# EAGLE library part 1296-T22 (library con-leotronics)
1.27mm SINGLE ROW FEMALE SOCKET Source: http://www.leotronics.co.uk/Conexcon/Data%20Sheets/sec.%20A/1296ing.pdf
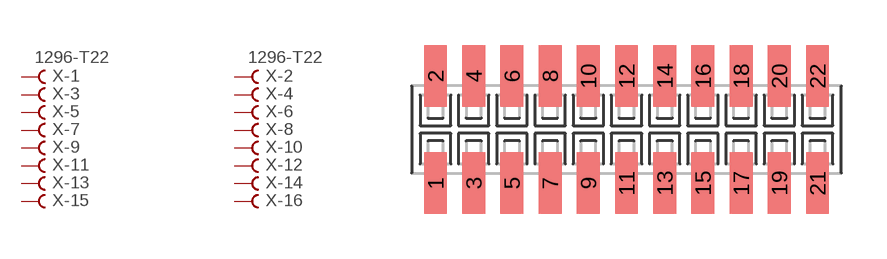
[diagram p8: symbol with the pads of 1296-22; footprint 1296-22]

Designator prefix X; gates -1=FVAL -2=FVAL -3=F -4=F -5=F -6=F -7=F -8=F -9=F -10=F -11=F -12=F -13=F -14=F -15=F -16=F -17=F -18=F -19=F -20=F -21=F -22=F

## 1296-T22 (OC_FARNELL: unknown; OC_NEWARK: unknown)  [1296-22]
1  -1:B  pas
2  -2:B  pas
3  -3:B  pas
4  -4:B  pas
5  -5:B  pas
6  -6:B  pas
7  -7:B  pas
8  -8:B  pas
9  -9:B  pas
10  -10:B  pas
11  -11:B  pas
12  -12:B  pas
13  -13:B  pas
14  -14:B  pas
15  -15:B  pas
16  -16:B  pas
17  -17:B  pas
18  -18:B  pas
19  -19:B  pas
20  -20:B  pas
21  -21:B  pas
22  -22:B  pas

## Footprint 1296-22 (pad centres in mm)
1.27mm SINGLE ROW FEMALE SOCKET Source: http://www.leotronics.co.uk/Conexcon/Data%20Sheets/sec.%20A/1296ing.pdf
smd 0.76 x 2.05: 1 -6.35,-1.78; 2 -6.35,1.78; 3 -5.08,-1.78; 4 -5.08,1.78; 5 -3.81,-1.78; 6 -3.81,1.78; 7 -2.54,-1.78; 8 -2.54,1.78; 9 -1.27,-1.78; 10 -1.27,1.78; 11 0,-1.78; 12 0,1.78; 13 1.27,-1.78; 14 1.27,1.78; 15 2.54,-1.78; 16 2.54,1.78; 17 3.81,-1.78; 18 3.81,1.78; 19 5.08,-1.78; 20 5.08,1.78; 21 6.35,-1.78; 22 6.35,1.78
